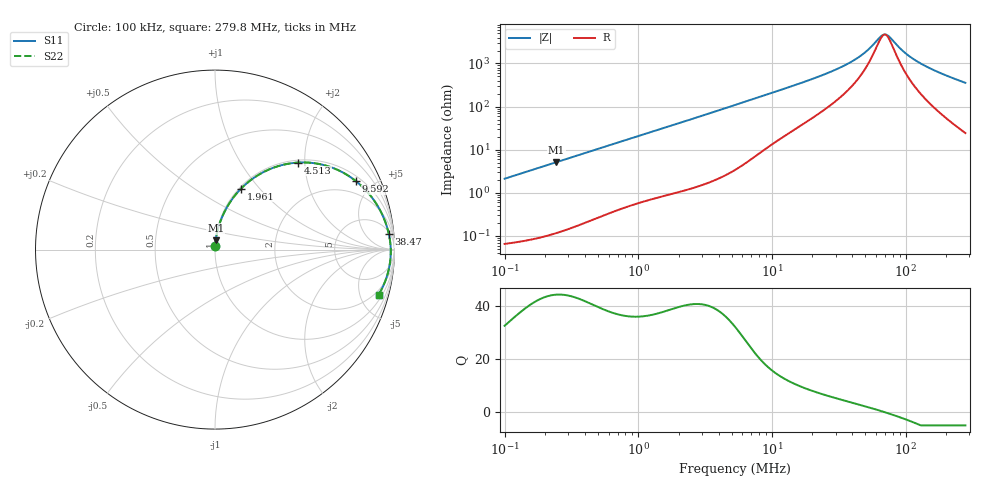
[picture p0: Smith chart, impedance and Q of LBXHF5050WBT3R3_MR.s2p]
! LBXHF5050WBT3R3_MR  S-PARAMETER MODEL  ( Standard Model )
! Model Generated by TAIYO YUDEN Corporation (http://www.ty-top.com)
! Version 1.0
! TAIYO YUDEN Control No. 220531
! Copyright(c) 2022 TAIYO YUDEN CO.,LTD. All Rights Reserved.
! Product Description (link to TY-COMPAS)
! https://ds.yuden.co.jp/TYCOMPAS/or/detail?pn=LBXHF5050WBT3R3NMR&u=M
! Products Name : Inductors
! Characteristics :
!  Inductance : 3.3 [uH] , SRF(min) : 55 [MHz] , DC Resistance(max) : 0.049 [Ohm]
!  Rated Current : Saturation  2500 [mA] , Temp Rise  1900 [mA]
!  Case Size : 5.0 x 5.0 / 0.197 x 0.197 [mm/inch] , Thickness : 2.2 / 0.087 [mm/inch]
!  (Conditions: Temperature = 25 [degC] , DC Bias Current = 0 [A])
! External Node Assignments :
!  1  o---GGG---o  2
! GND o---------o GND
! Frequency Range : 0.1MHz  -  279.750408MHz  [ 402 STEP ]
# MHz S RI R 50
! Freq[MHz].  S11 Real  S11 Imag  S21 Real  S21 Imag  S12 Real  S12 Imag  S22 Real  S22 Imag
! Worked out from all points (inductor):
!   401 points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, 100 kHz to 279.8 MHz, reference 50 ohm
!   read as one part in series: L = 3.38 uH near 104 kHz
!   highest Q = 44.2 at 244.2 kHz (marker M1), where L = 3.37 uH
!   self-resonance near 69.69 MHz
!   S11 on the Smith chart (normalised r, x): 100 kHz: 1.00, +0.04; 1.961 MHz: 1.02, +0.80; 4.513 MHz: 1.05, +1.85; 9.592 MHz: 1.24, +4.00; 38.47 MHz: 6, +20; 279.8 MHz: 1.49, -7.11
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0.1  0.0011 0.0212  0.9989 -0.0212  0.9989 -0.0212  0.0011 0.0212
0.244209  0.00382 0.0514  0.9962 -0.0514  0.9962 -0.0514  0.00382 0.0514
0.377863  0.00814 0.0788  0.9919 -0.0788  0.9919 -0.0788  0.00814 0.0788
0.756705  0.0283 0.1525  0.9717 -0.1525  0.9717 -0.1525  0.0283 0.1525
1.427803  0.0855 0.2666  0.9145 -0.2666  0.9145 -0.2666  0.0855 0.2666
1.961277  0.1454 0.34  0.8546 -0.34  0.8546 -0.34  0.1454 0.34
2.916605  0.2677 0.4306  0.7323 -0.4306  0.7323 -0.4306  0.2677 0.4306
4.51284  0.463 0.4849  0.537 -0.4849  0.537 -0.4849  0.463 0.4849
5.289144  0.5413 0.483  0.4587 -0.483  0.4587 -0.483  0.5413 0.483
9.591647  0.7867 0.3804  0.2133 -0.3804  0.2133 -0.3804  0.7867 0.3804
13.43943  0.8698 0.2963  0.1302 -0.2963  0.1302 -0.2963  0.8698 0.2963
19.9857  0.9272 0.2049  0.0728 -0.2049  0.0728 -0.2049  0.9272 0.2049
29.13675  0.9564 0.1322  0.0436 -0.1322  0.0436 -0.1322  0.9564 0.1322
38.46609  0.9687 0.0864  0.0313 -0.0864  0.0313 -0.0864  0.9687 0.0864
49.78495  0.9754 0.0478  0.0246 -0.0478  0.0246 -0.0478  0.9754 0.0478
67.04278  0.979 0.00546  0.021 -0.00546  0.021 -0.00546  0.979 0.00546
71.15457  0.9793 -0.00294  0.0207 0.00294  0.0207 0.00294  0.9793 -0.00294
75.51853  0.9793 -0.0114  0.0207 0.0114  0.0207 0.0114  0.9793 -0.0114
97.74029  0.9777 -0.0489  0.0223 0.0489  0.0223 0.0489  0.9777 -0.0489
124.0157  0.9729 -0.0862  0.0271 0.0862  0.0271 0.0862  0.9729 -0.0862
177.248  0.9574 -0.1501  0.0426 0.1501  0.0426 0.1501  0.9574 -0.1501
279.7504  0.9122 -0.2508  0.0878 0.2508  0.0878 0.2508  0.9122 -0.2508
